FUNCTION "ComunicazioneOp" : VOID
TITLE =Comunicazioni con op
VERSION : 0.1

BEGIN
NETWORK
TITLE =Controllo Arrivo Set Di dati
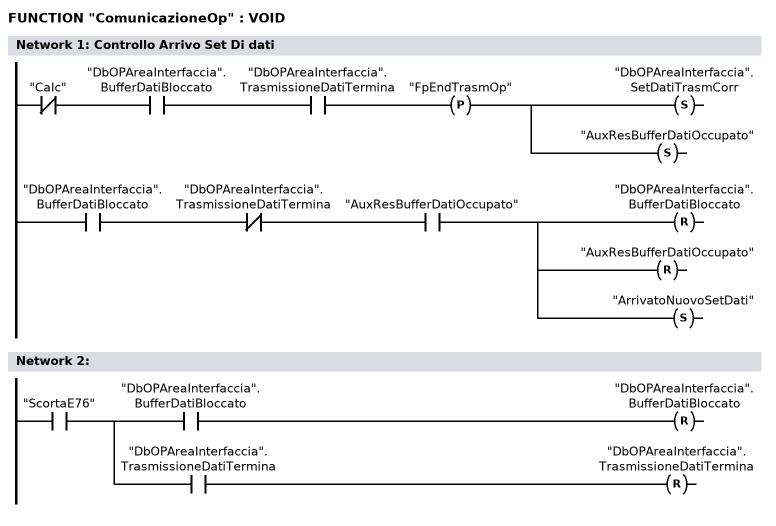
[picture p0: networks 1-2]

      UN    "CaIc";
      U     "DbOPAreaInterfaccia".BufferDatiBloccato;
      U     "DbOPAreaInterfaccia".TrasmissioneDatiTermina;
      FP    "FpEndTrasmOp";
      S     "DbOPAreaInterfaccia".SetDatiTrasmCorr;
      S     "AuxResBufferDatiOccupato";


      U     "DbOPAreaInterfaccia".BufferDatiBloccato;
      UN    "DbOPAreaInterfaccia".TrasmissioneDatiTermina;
      U     "AuxResBufferDatiOccupato";
      R     "DbOPAreaInterfaccia".BufferDatiBloccato;
      R     "AuxResBufferDatiOccupato";
      S     "ArrivatoNuovoSetDati";


NETWORK
TITLE =

      U     "ScortaE76";
      =     L      0.0;
      U     L      0.0;
      U     "DbOPAreaInterfaccia".BufferDatiBloccato;
      R     "DbOPAreaInterfaccia".BufferDatiBloccato;
      U     L      0.0;
      U     "DbOPAreaInterfaccia".TrasmissioneDatiTermina;
      R     "DbOPAreaInterfaccia".TrasmissioneDatiTermina;
END_FUNCTION

